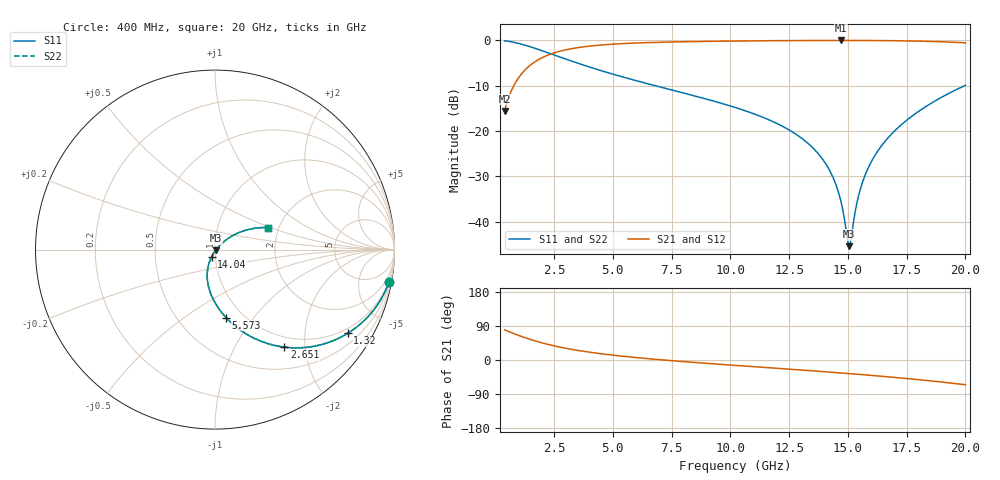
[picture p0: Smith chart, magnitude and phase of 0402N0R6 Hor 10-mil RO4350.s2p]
# GHz S MA R 50
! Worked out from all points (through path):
!   1960 points, 400 MHz to 20 GHz, reference 50 ohm
!   highest |S21| = -0.05 dB at 14.7 GHz (marker M1); lowest = -15.6 dB at 400 MHz (marker M2)
!   lowest |S11| = -45.4 dB at 15.06 GHz (marker M3), VSWR 1.01, Z = 50.4 - j0.33 ohm
!   |S11| at or under -10 dB: 6.783 GHz to 19.98 GHz (13.2 GHz wide, 98.6 % of centre)
!   |S22| runs from -45.4 to -0.1 dB; largest |S21 - S12| = 0
!   S11 on the Smith chart (normalised r, x): 400 MHz: 1, -11; 1.32 GHz: 0.83, -3.27; 2.651 GHz: 0.83, -1.62; 5.573 GHz: 0.83, -0.74; 14.04 GHz: 0.96, -0.08; 20 GHz: 1.75, +0.48
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0.4  0.9862 -10.5  0.1655 79.5  0.1655 79.5  0.9862 -10.5
0.8102093  0.9467 -20.8  0.3218 69.2  0.3218 69.2  0.9467 -20.8
1.32047  0.8744 -32.2  0.4847 57.7  0.4847 57.7  0.8744 -32.2
2.651149  0.6668 -54.6  0.7442 35.3  0.7442 35.3  0.6668 -54.6
3.671669  0.5408 -66.1  0.8398 23.8  0.8398 23.8  0.5408 -66.1
5.572639  0.3838 -80.8  0.9215 9.0  0.9215 9.0  0.3838 -80.8
6.943338  0.3084 -88.5  0.9489 1.1  0.9489 1.1  0.3084 -88.5
10.205  0.1814 -103.2  0.98 -14.2  0.98 -14.2  0.1814 -103.2
12.166  0.1143 -110.8  0.9892 -22.7  0.9892 -22.7  0.1143 -110.8
13.46667  0.06675 -114.6  0.9928 -28.4  0.9928 -28.4  0.06675 -114.6
14.03696  0.0443 -114.9  0.9937 -31.0  0.9937 -31.0  0.0443 -114.9
14.41715  0.02871 -112.9  0.9941 -32.8  0.9941 -32.8  0.02871 -112.9
14.69729  0.01702 -106.6  0.9941 -34.1  0.9941 -34.1  0.01702 -106.6
14.97744  0.006521 -71.1  0.9941 -35.5  0.9941 -35.5  0.006521 -71.1
15.05748  0.005359 -37.7  0.994 -35.8  0.994 -35.8  0.005359 -37.7
15.13752  0.006443 -3.4  0.994 -36.2  0.994 -36.2  0.006443 -3.4
15.42767  0.01799 34.1  0.9936 -37.7  0.9936 -37.7  0.01799 34.1
15.69781  0.03075 40.0  0.9931 -39.0  0.9931 -39.0  0.03075 40.0
16.13803  0.05292 42.0  0.9918 -41.3  0.9918 -41.3  0.05292 42.0
16.73834  0.08552 41.0  0.9889 -44.5  0.9889 -44.5  0.08552 41.0
18.10904  0.1711 34.8  0.9763 -52.5  0.9763 -52.5  0.1711 34.8
20  0.3181 22.7  0.9363 -65.3  0.9363 -65.3  0.3181 22.7
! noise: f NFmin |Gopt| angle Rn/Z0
0.4  0.001427  0.8594  6.496  0.002165
2.571  0.004674  0.6666  10.88  0.002666
4.752  0.007484  0.6189  14.96  0.003602
6.933  0.01022  0.5977  19.4  0.004548
9.104  0.01307  0.5907  23.88  0.005613
11.29  0.01624  0.5942  28.34  0.006933
13.47  0.01993  0.6068  32.72  0.008678
15.64  0.02443  0.6277  36.99  0.01112
17.82  0.03025  0.6569  41.22  0.01482
20  0.03821  0.6942  45.44  0.02086
